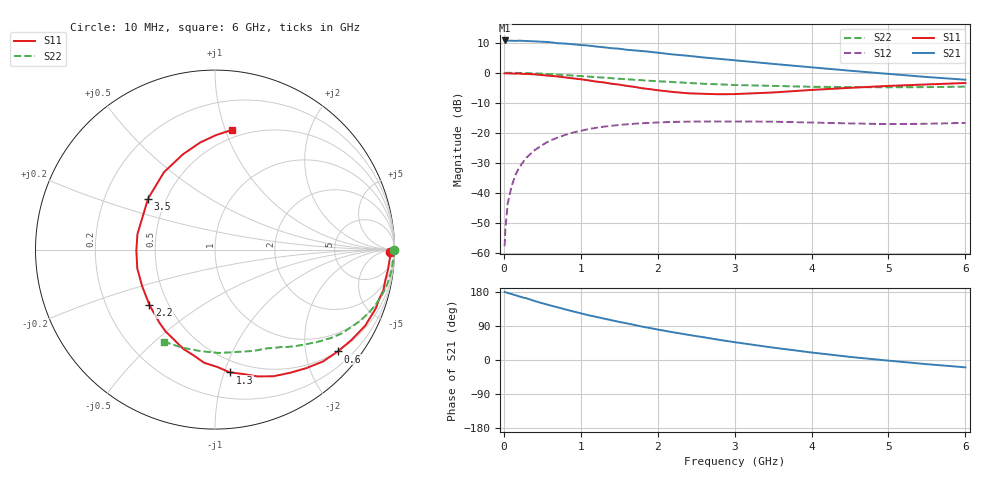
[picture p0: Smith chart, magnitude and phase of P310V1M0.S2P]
! SIEMENS Small Signal Semiconductors
! BFP181
! Si NPN RF Bipolar Junction Transistor in SOT143
! VCE = 10 V  IC = 1 mA
! Common Emitter S-Parameters:  March  1996
# GHz  S  MA  R  50
!  f  S11  S21  S12  S22
! GHz  MAG  ANG  MAG  ANG  MAG  ANG  MAG  ANG
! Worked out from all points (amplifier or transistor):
!   36 points, 10 MHz to 6 GHz, reference 50 ohm
!   highest |S21| = 10.7 dB at 10 MHz (marker M1)
!   |S21| within 3 dB of that: start of sweep to 1.571 GHz
!   unconditionally stable (mu >= 1): 3.293 GHz to end of sweep
!   at 250 MHz: K = 0.09, MSG = 20.2 dB, |S12| = -29.7 dB
!   at 1.4 GHz: K = 0.48, MSG = 12.9 dB, |S12| = -17.7 dB
!   at 6 GHz: K = 1.28, MAG = 4.0 dB, |S12| = -16.7 dB
!   S11 on the Smith chart (normalised r, x): 10 MHz: 61, -34; 600 MHz: 0.50, -2.69; 1.3 GHz: 0.40, -1.05; 2.2 GHz: 0.39, -0.31; 3.5 GHz: 0.40, +0.29; 6 GHz: 0.43, +1.06
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0.01  0.9755 -0.8  3.439 179.4  0.0013 86.2  0.9983 -0.2
0.02  0.9774 -1.1  3.409 179.2  0.0025 84.2  0.9917 -0.6
0.05  0.9751 -3.0  3.413 177.0  0.0066 90.8  0.9958 -1.7
0.1  0.9698 -7.0  3.404 174.1  0.0128 85.8  0.9943 -3.2
0.15  0.9646 -9.9  3.384 171.0  0.0198 82.6  0.9925 -4.8
0.2  0.965 -13.6  3.415 167.8  0.0264 80.2  0.9907 -6.5
0.3  0.954 -20.1  3.359 162.5  0.0394 76.6  0.9834 -9.7
0.4  0.9381 -26.9  3.324 155.7  0.0513 72.3  0.9745 -12.8
0.6  0.8887 -39.7  3.22 144.3  0.0741 63.6  0.9467 -18.8
0.8  0.8336 -52.4  3.048 133.5  0.0926 55.7  0.9142 -24.1
1.1  0.7461 -71.3  2.827 118.2  0.1151 45.1  0.8607 -31.3
1.3  0.6892 -83.1  2.646 109.3  0.1264 38.9  0.8269 -35.6
1.5  0.6335 -95.5  2.506 100.5  0.135 33.7  0.7915 -39.3
1.8  0.5503 -114.7  2.291 88.0  0.1444 27.0  0.7484 -44.1
2.2  0.4779 -139.9  2.01 73.2  0.1518 19.0  0.6983 -50.4
2.4  0.454 -153.5  1.91 66.3  0.1534 15.6  0.6761 -53.4
2.8  0.4382 -179.6  1.699 53.2  0.1542 10.2  0.64 -58.9
3.5  0.4689 142.7  1.401 32.7  0.1532 2.7  0.6036 -69.3
4  0.5166 123.4  1.229 19.8  0.1481 -0.4  0.5829 -78.0
4.5  0.5603 108.6  1.079 8.2  0.1434 -2.8  0.5763 -87.8
5.5  0.6379 89.5  0.848 -11.0  0.1414 -1.1  0.5755 -108.1
6  0.6738 81.9  0.764 -19.4  0.1464 -0.5  0.5865 -118.8
